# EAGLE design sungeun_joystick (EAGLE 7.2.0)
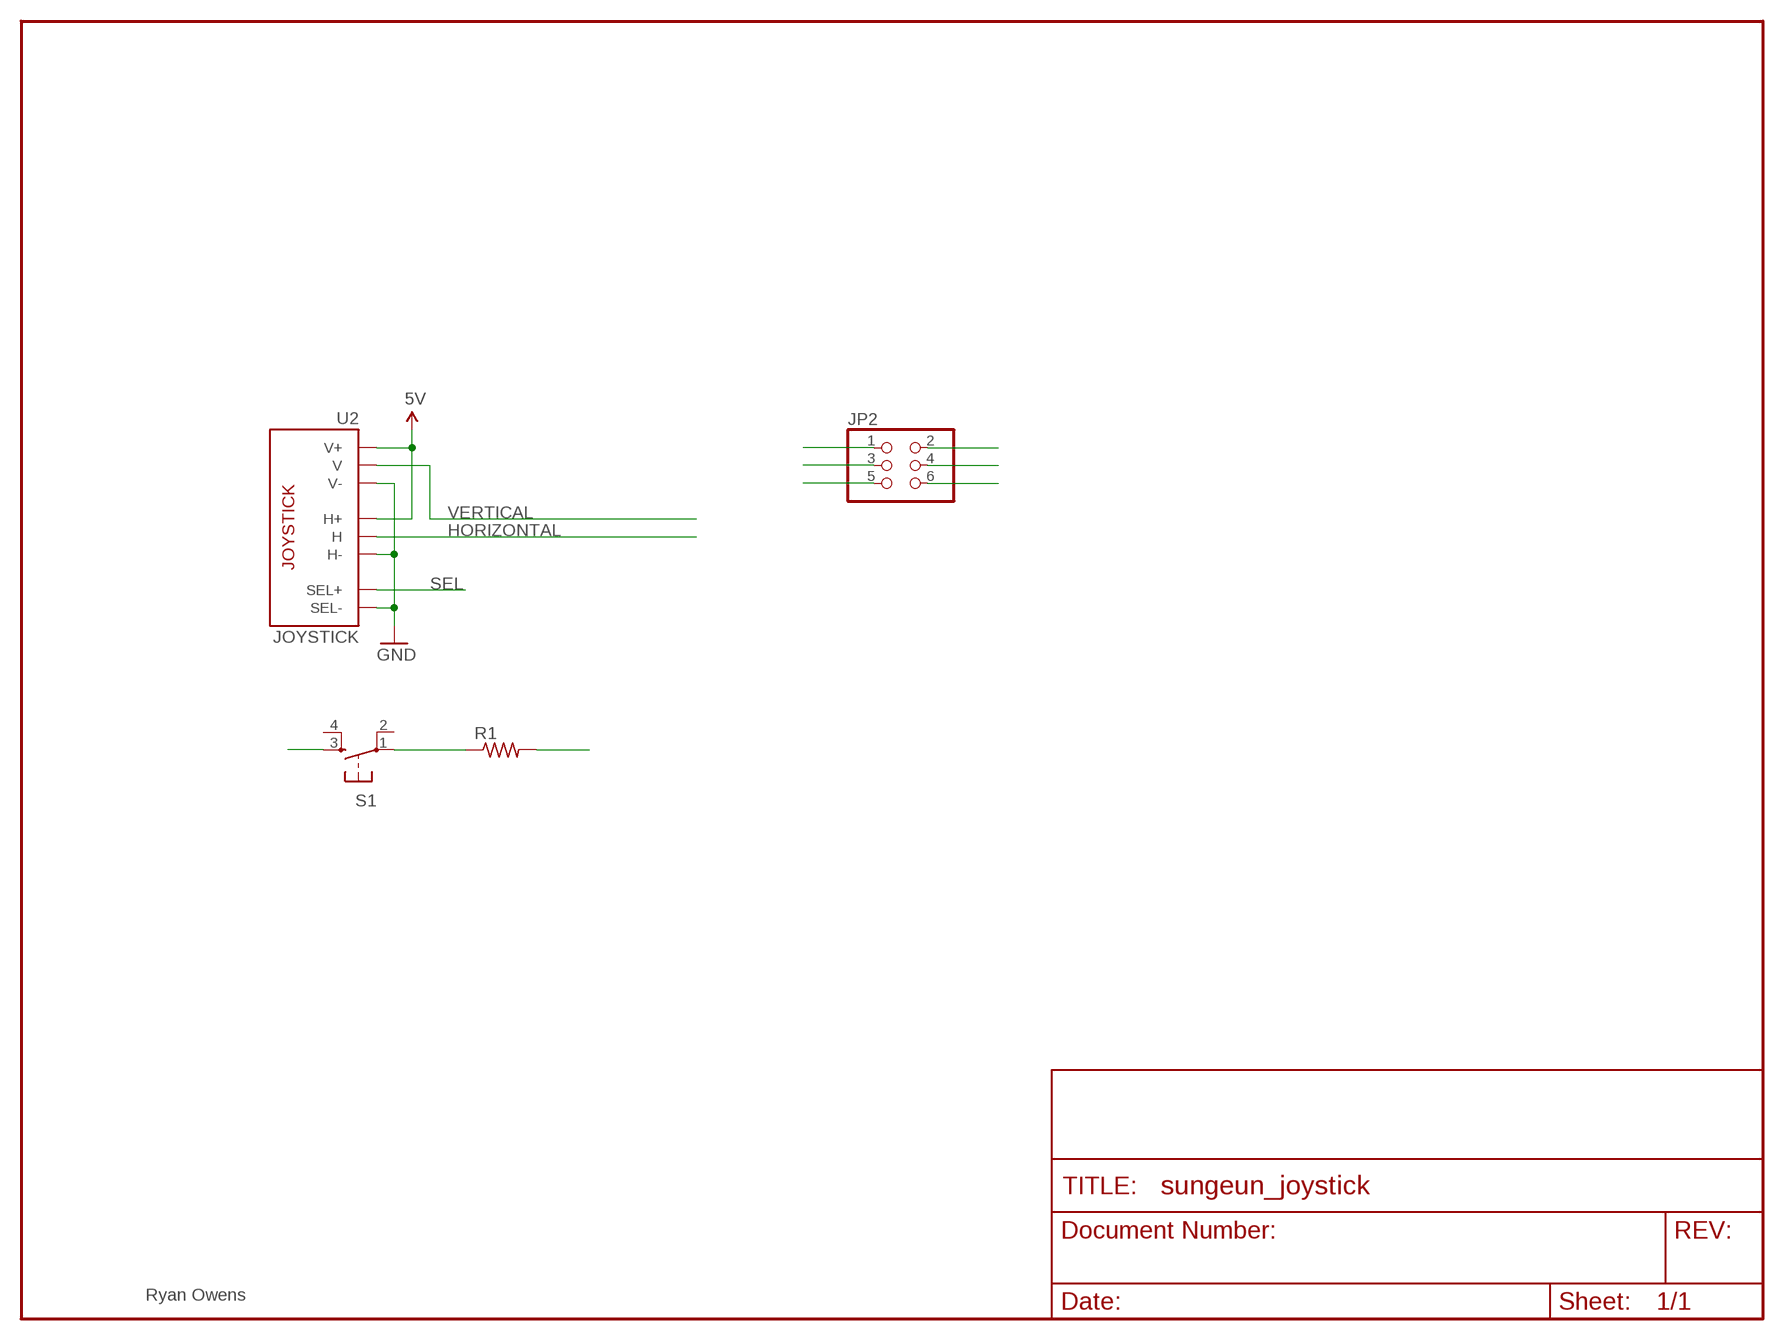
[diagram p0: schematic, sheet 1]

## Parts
JP2  PINHD-2X3-SMD  [2X03SMD]
R1  RESISTOR1206  [1206]
S1  6MM_SWITCH6MM_SWITCH  [6MM_SWITCH]
U2  JOYSTICK  JOYSTICKPTH  [JOYSTICK]

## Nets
5V: JP2.1 R1.2 U2.H1(H+) U2.V1(V+)
GND: JP2.2 S1.3(S) U2.B2A(SEL-) U2.H3(H-) U2.V3(V-)
HORIZONTAL: JP2.5 U2.H2(H)
MODE: JP2.6 R1.1 S1.1(P)
SEL: JP2.4 U2.B1A(SEL+)
VERTICAL: JP2.3 U2.V2(V)
Unconnected: S1.2(P1) S1.4(S1)

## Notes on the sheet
- Ryan Owens

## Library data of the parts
JP2 = fab:PINHD-2X3-SMD: PIN HEADER
R1 = ng:RESISTOR
S1 = fab:6MM_SWITCH: OMRON SWITCH
U2 = SparkFun:JOYSTICK: Thumb Joystick Joystick commonly found in PS2 controllers. Two pots and a select switch. Footprint proven. Spark Fun Electronics SKU : COM-09032

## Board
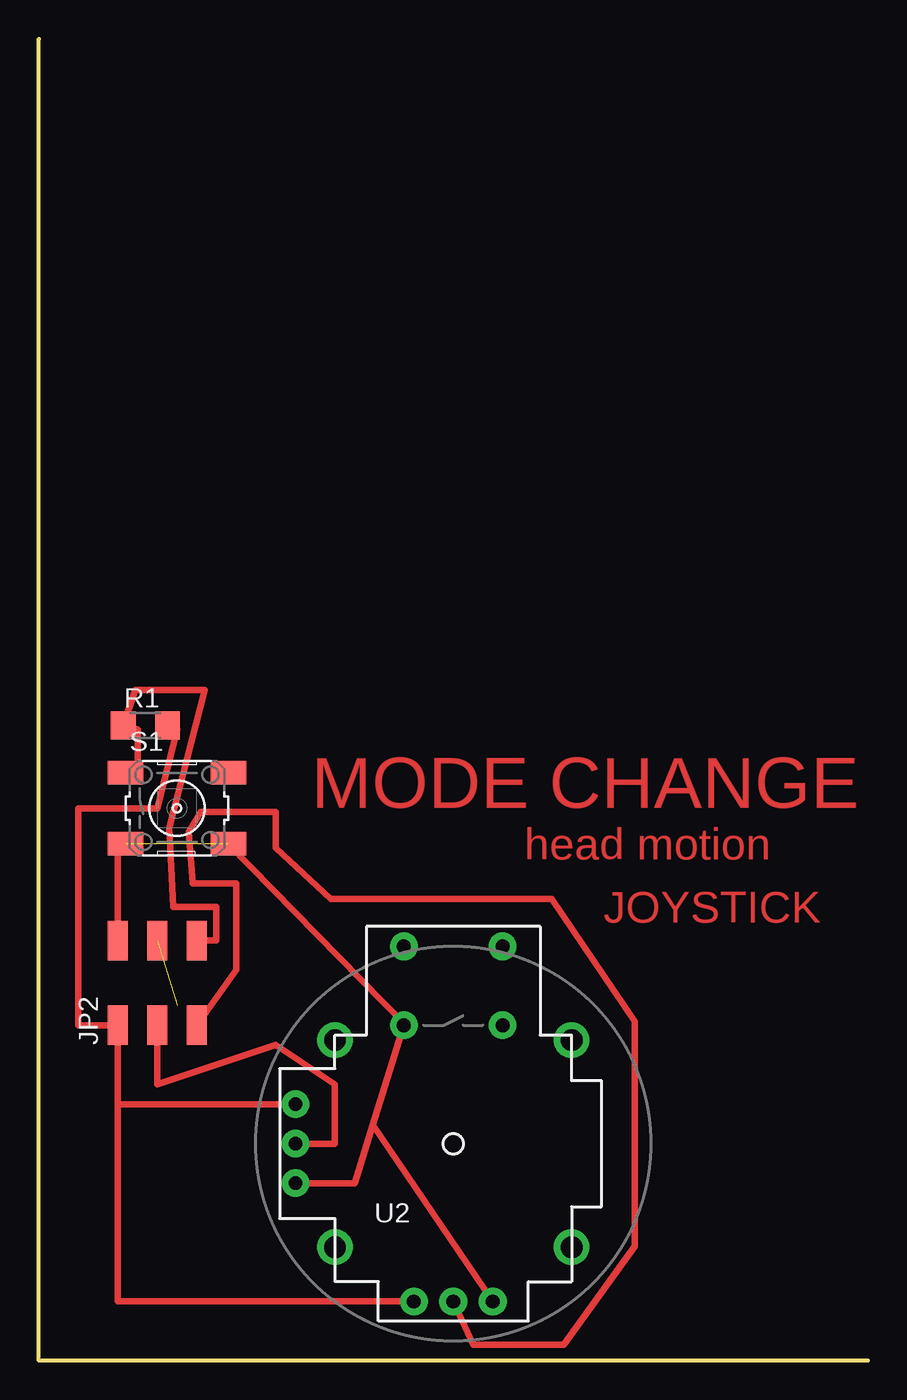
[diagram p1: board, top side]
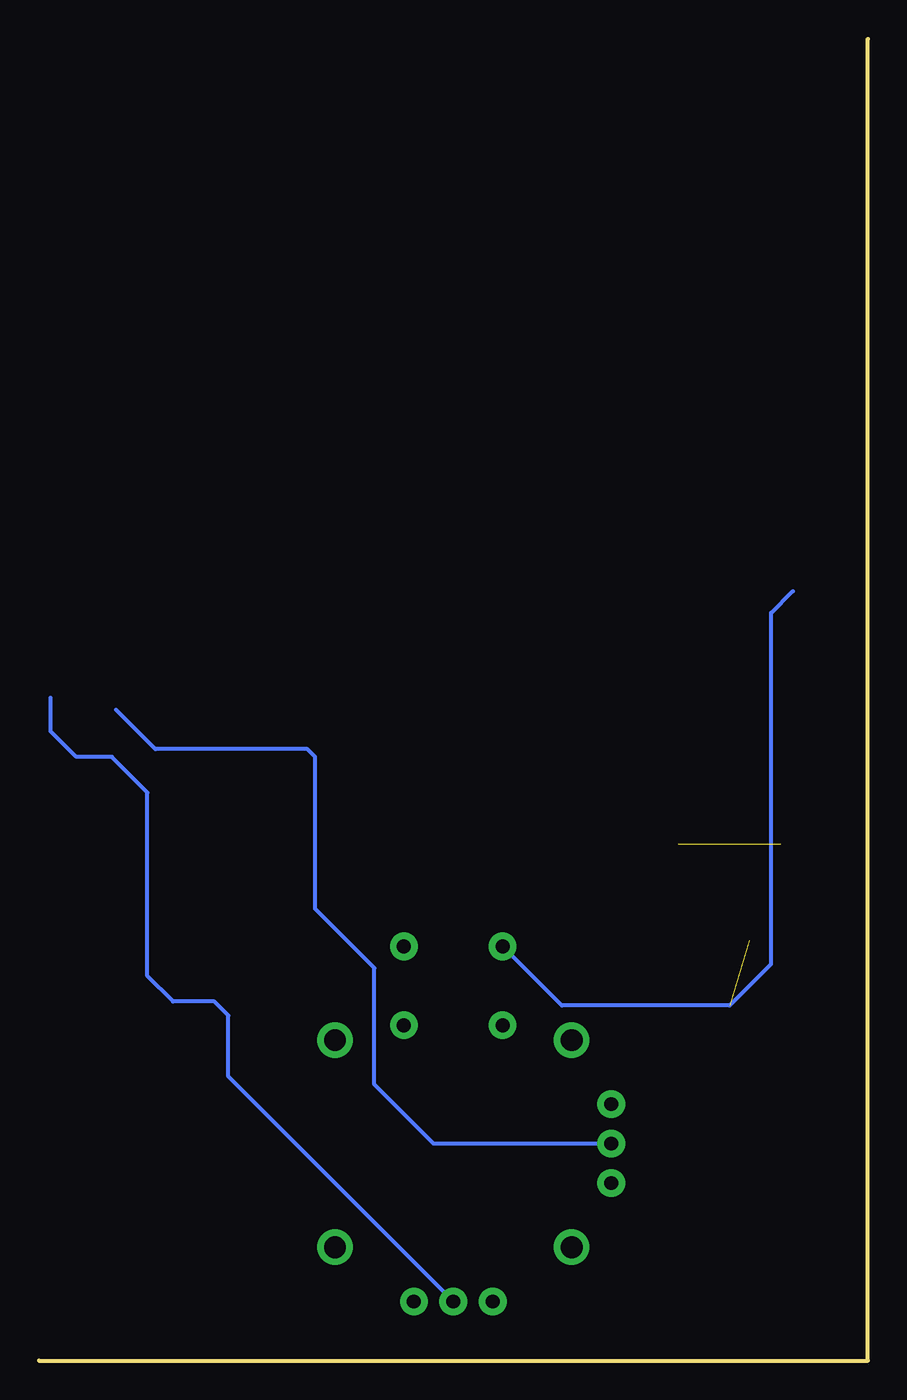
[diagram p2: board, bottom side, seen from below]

Size 53.34 x 85.09 mm. Coordinates in mm from the lower left corner, seen from the top.
Outline: 0,85.09 0,0 53.34,0
Copper layers (1*16): Top 0.035mm / dielectric 1.5mm / Bottom 0.035mm
Design rules "SparkFun": minimum track width 8mil, minimum drill 20mil, track to track 8mil, track to pad 8mil, pad to pad 8mil, via to via 8mil, smd to smd 8mil, copper to edge 9mil, drill to drill 8mil, minimum pad ring 12mil, minimum via ring 10mil, stop-mask expansion 4mil, vias tented up to drill 20mil, thermal gap 10mil

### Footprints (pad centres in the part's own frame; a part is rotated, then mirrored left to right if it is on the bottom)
2X03SMD = smd 2.54 x 1.27: 1 -2.54,2.54; 2 2.92,2.54; 3 -2.54,0; 4 2.92,0; 5 -2.54,-2.54; 6 2.92,-2.54
1206 = smd 1.6 x 1.803: 1 -1.422,0; 2 1.422,0
6MM_SWITCH = smd 2.286 x 1.524: 1 -3.302,2.286; 2 3.302,2.286; 3 -3.302,-2.286; 4 3.302,-2.286
JOYSTICK = drill 0.9 pad 1.778: B1A -3.175,12.7; B1B 3.175,12.7; B2A -3.175,7.62; B2B 3.175,7.62 | drill 0.889 pad 1.778: H1 -2.54,-10.16; H2 0,-10.16; H3 2.54,-10.16; V1 -10.16,2.54; V2 -10.16,0; V3 -10.16,-2.54 | drill 1.397 pad 2.286: MOUNT1 -7.62,6.668; MOUNT2 -7.62,-6.668; MOUNT3 7.62,-6.668; MOUNT4 7.62,6.668

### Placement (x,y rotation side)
JP2  7.62,24.13 90 top
R1  6.86,40.89 0 top
S1  8.89,35.56 0 top
U2  26.67,13.97 0 top

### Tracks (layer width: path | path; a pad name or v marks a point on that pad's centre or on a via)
5V
  Top 0.406: R1.2 8.89,40.64 7.62,35.56 2.54,35.56 2.54,21.59 JP2.1 5.08,16.51 | 5.08,16.51 U2.V1 | U2.H1 5.08,3.81 5.08,16.51
GND  (1 unrouted)
  Top 0.406: S1.3 5.08,33.27 JP2.2 | U2.V3 20.32,11.43 21.5,15.19 | 21.5,15.19 U2.B2A 23.62,21.59 12.19,33.27 | U2.H3 21.5,15.19
HORIZONTAL
  Top 0.406: U2.H2 27.94,1.02 33.78,1.02 38.35,7.37 38.35,21.84 33.02,29.72 18.8,29.72 15.24,33.02 15.24,35.31 10.41,35.31 9.65,34.04 9.91,30.73 12.7,30.73 12.7,25.15 JP2.5
  Bottom 0.254: U2.H2 41.15,18.29 41.15,22.23 42.04,23.11 44.7,23.11 46.35,24.77 46.35,36.58 48.64,38.86 50.93,38.86 52.58,40.51 52.58,42.67
MODE
  Top 0.406: S1.1 6.35,37.85 6.35,40.64 R1.1 6.2,43.18 10.67,43.18 8.38,34.29 8.64,29.21 11.43,29.21 11.43,27.05 JP2.6
SEL  (1 unrouted)
  Bottom 0.254: 4.83,49.53 6.22,48.13 6.22,25.53 8.89,22.86 19.68,22.86 U2.B1A
VERTICAL
  Top 0.406: U2.V2 19.05,13.97 19.05,17.78 15.24,20.32 7.62,17.78 JP2.3
  Bottom 0.254: U2.V2 27.94,13.97 31.75,17.78 31.75,25.27 35.56,29.08 35.56,38.86 36.07,39.37 45.85,39.37 48.39,41.91

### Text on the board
Top: MODE CHANGE | head motion | JOYSTICK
